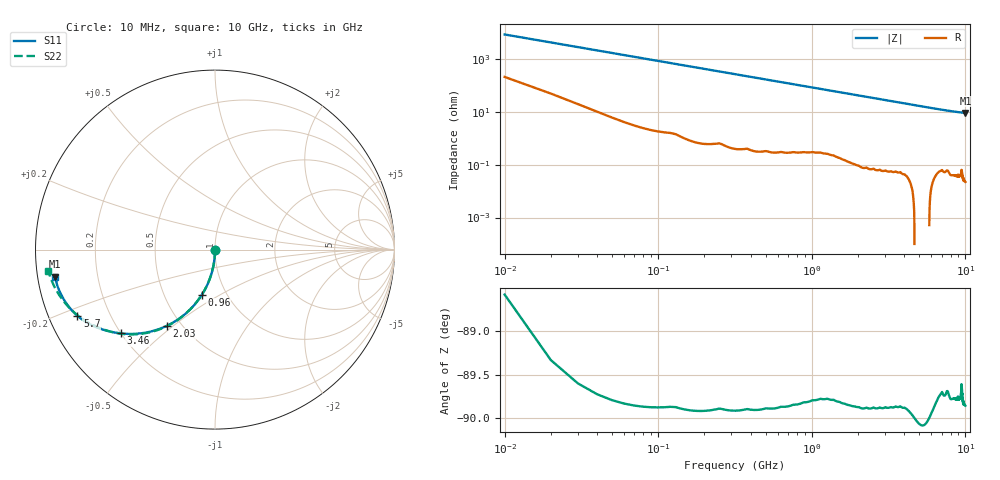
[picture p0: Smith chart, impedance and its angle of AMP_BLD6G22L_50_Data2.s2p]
! Created Fri Sep 09 16:28:08 2011
# ghz S ma R 50
! 2 Port Network Data from SP1.SP block
! freq  magS11  angS11  magS21  angS21  magS12  angS12  magS22  angS22
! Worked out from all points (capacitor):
!   1000 points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, 10 MHz to 10 GHz, reference 50 ohm
!   read as one part in shunt: C = 1.88 pF near 60 MHz
!   lowest |Z| = 9.02 ohm at 10 GHz (marker M1)
!   S11 on the Smith chart (normalised r, x): 10 MHz: 1.00, -0.01; 960 MHz: 0.76, -0.42; 2.03 GHz: 0.42, -0.47; 3.46 GHz: 0.20, -0.37; 5.7 GHz: 0.08, -0.23; 10 GHz: 0.05, -0.08
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0.01  0.002869 -91.8  0.9999 -0.2  0.9999 -0.2  0.002883 -91.3
0.04  0.01147 -91.0  0.9999 -0.7  0.9999 -0.7  0.01153 -90.9
0.07  0.02007 -91.3  0.9997 -1.2  0.9997 -1.2  0.02018 -91.4
0.1  0.02867 -91.8  0.9995 -1.7  0.9995 -1.7  0.02882 -91.9
0.13  0.03726 -92.4  0.9992 -2.3  0.9992 -2.3  0.03745 -92.4
0.16  0.04584 -92.8  0.9989 -2.8  0.9989 -2.8  0.04608 -92.9
0.24  0.06867 -94.2  0.9975 -4.2  0.9975 -4.2  0.06903 -94.3
0.36  0.1027 -96.3  0.9945 -6.2  0.9945 -6.2  0.1032 -96.4
0.52  0.1475 -99.0  0.9887 -9.0  0.9887 -9.0  0.1483 -99.1
0.72  0.2023 -102.4  0.9787 -12.3  0.9787 -12.3  0.2032 -102.5
0.96  0.2655 -106.4  0.963 -16.3  0.963 -16.3  0.2664 -106.5
1.29  0.347 -111.6  0.9363 -21.5  0.9363 -21.5  0.3472 -111.7
1.68  0.434 -117.5  0.8992 -27.3  0.8992 -27.3  0.4345 -117.4
2.03  0.503 -122.3  0.8623 -32.1  0.8623 -32.1  0.5044 -122.1
2.64  0.6032 -129.9  0.7943 -39.8  0.7943 -39.8  0.6058 -129.8
3.34  0.6909 -137.3  0.7175 -47.3  0.7175 -47.3  0.6942 -137.3
3.46  0.7035 -138.4  0.7048 -48.4  0.7048 -48.4  0.7068 -138.5
5.01  0.8209 -150.3  0.5645 -60.8  0.5645 -60.8  0.8227 -151.0
5.7  0.851 -154.3  0.515 -64.9  0.515 -64.9  0.8552 -155.4
6.67  0.8765 -159.1  0.4574 -69.6  0.4574 -69.6  0.887 -160.5
8.34  0.898 -165.5  0.386 -76.2  0.386 -76.2  0.9194 -167.3
10  0.9047 -170.4  0.3411 -81.5  0.3411 -81.5  0.9362 -172.7
